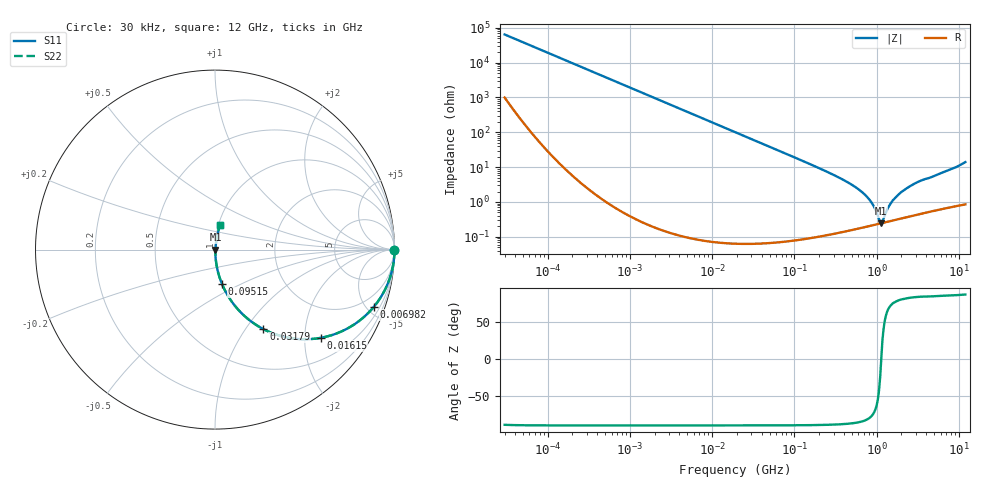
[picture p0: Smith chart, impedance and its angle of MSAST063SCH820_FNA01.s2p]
! MSAST063SCH820_FNA01  S-PARAMETER MODEL  ( Standard Model )
! Model Generated by TAIYO YUDEN Corporation (http://www.ty-top.com)
! Version 1.0
! TAIYO YUDEN Control No. 241122
! Copyright(c) 2024 TAIYO YUDEN CO.,LTD. All Rights Reserved.
! Product Description (link to TY-COMPAS)
! https://ds.yuden.co.jp/TYCOMPAS/or/detail?pn=MSAST063SCH820JFNA01&u=M
! Products Name : Multilayer Ceramic Capacitors
! Characteristics :
!  Capacitance : 82 [pF] , Rated Voltage : 25 [V] , TCC : CH / C0H
!  Case Size : 0.6 x 0.3 / 0.024 x 0.012 [mm/inch] , Thickness : 0.3 / 0.012 [mm/inch]
!  (Conditions: Temperature = 25 [degC] , DC Bias Voltage = 0 [V])
! External Node Assignments :
!  1  o---| |---o  2
! GND o---------o GND
! Frequency Range : 0.03MHz  -  12000MHz  [ 401 STEP ]
# MHZ S RI R 50
! Freq[MHz].  S11 Real  S11 Imag  S21 Real  S21 Imag  S12 Real  S12 Imag  S22 Real  S22 Imag
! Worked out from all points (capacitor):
!   401 points, 30 kHz to 12 GHz, reference 50 ohm
!   read as one part in series: C = 82.4 pF near 32 kHz
!   lowest |Z| = 245 mohm at 1.14 GHz (marker M1)
!   series resonance near 1.139 GHz, so ESL is about 240 pH
!   S11 on the Smith chart (normalised r, x): 30 kHz: open; 6.982 MHz: 1.00, -5.53; 16.15 MHz: 1.00, -2.39; 31.79 MHz: 1.00, -1.21; 95.15 MHz: 1.00, -0.40; 12 GHz: 1.02, +0.28
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0.03  1 -0.00155  2.65e-05 0.00155  2.65e-05 0.00155  1 -0.00155
0.260295  0.9998 -0.0135  0.000188 0.0135  0.000188 0.0135  0.9998 -0.0135
2.258455  0.9865 -0.1154  0.0135 0.1154  0.0135 0.1154  0.9865 -0.1154
6.982189  0.8843 -0.3197  0.1157 0.3197  0.1157 0.3197  0.8843 -0.3197
10.61839  0.7677 -0.4221  0.2323 0.4221  0.2323 0.4221  0.7677 -0.4221
16.14825  0.5883 -0.4919  0.4117 0.4919  0.4117 0.4919  0.5883 -0.4919
18.97367  0.5086 -0.4996  0.4914 0.4996  0.4914 0.4996  0.5086 -0.4996
31.78584  0.2695 -0.4432  0.7305 0.4432  0.7305 0.4432  0.2695 -0.4432
53.24956  0.1162 -0.3196  0.8838 0.3196  0.8838 0.3196  0.1162 -0.3196
95.14999  0.0397 -0.1934  0.9603 0.1934  0.9603 0.1934  0.0397 -0.1934
164.6252  0.0139 -0.1131  0.9861 0.1131  0.9861 0.1131  0.0139 -0.1131
380.7415  0.00338 -0.0449  0.9966 0.0449  0.9966 0.0449  0.00338 -0.0449
637.8412  0.00221 -0.0207  0.9978 0.0207  0.9978 0.0207  0.00221 -0.0207
852.6267  0.00218 -0.00996  0.9978 0.00996  0.9978 0.00996  0.00218 -0.00996
939.2353  0.00224 -0.0066  0.9978 0.0066  0.9978 0.0066  0.00224 -0.0066
1068.55  0.00237 -0.00221  0.9976 0.00221  0.9976 0.00221  0.00237 -0.00221
1139.739  0.00245 3.63e-05  0.9976 -3.63e-05  0.9976 -3.63e-05  0.00245 3.63e-05
1215.67  0.00254 0.00217  0.9975 -0.00217  0.9975 -0.00217  0.00254 0.00217
1428.372  0.00284 0.00736  0.9972 -0.00736  0.9972 -0.00736  0.00284 0.00736
1848.769  0.00347 0.016  0.9965 -0.016  0.9965 -0.016  0.00347 0.016
2722.352  0.00494 0.0306  0.9951 -0.0306  0.9951 -0.0306  0.00494 0.0306
12000  0.0272 0.1349  0.9728 -0.1349  0.9728 -0.1349  0.0272 0.1349
